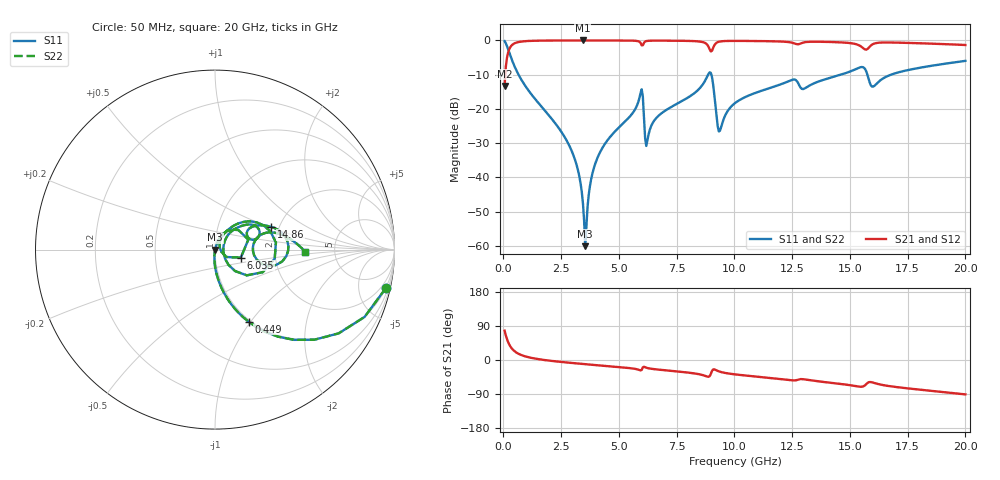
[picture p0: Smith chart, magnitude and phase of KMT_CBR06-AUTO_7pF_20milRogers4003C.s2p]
! Data measured by Modelithics Inc. support@modelithics.com 813-866-6335
! KEMET CBR06-AUTO 7pF, Pad Width= 0.851mm, Pad Length= 0.64mm, Pad Gap= 0.62mm, 20mil Rogers 4003C substrate Data, January 2022
# hz S ma R 50
! 2 Port Network Data from SP1.SP block
! freq  magS11  angS11  magS21  angS21  magS12  angS12  magS22  angS22
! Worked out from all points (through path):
!   401 points, 50 MHz to 20 GHz, reference 50 ohm
!   highest |S21| = -0.01 dB at 3.442 GHz (marker M1); lowest = -13.3 dB at 50 MHz (marker M2)
!   group delay of S21, straight-line fit = 14 ps
!   lowest |S11| = -60.1 dB at 3.541 GHz (marker M3), VSWR 1.00, Z = 50.1 - j0.0405 ohm
!   |S11| at or under -10 dB: 654 MHz to 8.861 GHz (8.207 GHz wide, 173 % of centre); 9.001 GHz to 14.6 GHz (5.601 GHz wide, 47.5 % of centre); 15.76 GHz to 16.78 GHz (1.024 GHz wide, 6.29 % of centre)
!   |S22| runs from -60.1 to -0.2 dB; largest |S21 - S12| = 0
!   S11 on the Smith chart (normalised r, x): 50 MHz: 0.98, -8.90; 449 MHz: 0.98, -0.98; 6.035 GHz: 1.33, -0.12; 14.86 GHz: 1.82, +0.52; 20 GHz: 3.02, -0.10
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5e7  0.9762 -12.7  0.2167 77.3  0.2167 77.3  0.9762 -12.7
4.49e8  0.4429 -65.0  0.896 24.9  0.896 24.9  0.4429 -65.0
2.793125e9  0.03186 -95.4  0.9985 -6.9  0.9985 -6.9  0.03186 -95.4
3.192125e9  0.01418 -95.5  0.9989 -9.2  0.9989 -9.2  0.01418 -95.5
3.391625e9  0.006126 -91.4  0.9989 -10.2  0.9989 -10.2  0.006126 -91.4
3.4415e9  0.004198 -87.4  0.9989 -10.5  0.9989 -10.5  0.004198 -87.4
3.54125e9  0.0009928 -24.0  0.9989 -11.0  0.9989 -11.0  0.0009928 -24.0
3.8405e9  0.01103 72.1  0.9988 -12.6  0.9988 -12.6  0.01103 72.1
4.189625e9  0.02361 72.9  0.9985 -14.4  0.9985 -14.4  0.02361 72.9
5.93525e9  0.1702 39.8  0.9219 -27.5  0.9219 -27.5  0.1702 39.8
6.035e9  0.1505 -17.3  0.8493 -19.0  0.8493 -19.0  0.1505 -17.3
6.2345e9  0.03489 44.0  0.9847 -21.2  0.9847 -21.2  0.03489 44.0
6.73325e9  0.08061 62.1  0.9932 -25.6  0.9932 -25.6  0.08061 62.1
8.92775e9  0.3419 6.7  0.7429 -42.7  0.7429 -42.7  0.3419 6.7
9.32675e9  0.04689 -6.1  0.9566 -29.9  0.9566 -29.9  0.04689 -6.1
1.0025e10  0.1216 48.4  0.9844 -37.9  0.9844 -37.9  0.1216 48.4
1.336662e10  0.2301 31.7  0.9569 -54.3  0.9569 -54.3  0.2301 31.7
1.486288e10  0.3378 22.0  0.9245 -65.2  0.9245 -65.2  0.3378 22.0
1.576062e10  0.3128 -16.9  0.7496 -60.6  0.7496 -60.6  0.3128 -16.9
1.601e10  0.2119 3.9  0.8873 -59.8  0.8873 -59.8  0.2119 3.9
1.670825e10  0.3096 17.9  0.9334 -68.9  0.9334 -68.9  0.3096 17.9
2e10  0.5029 -1.4  0.8575 -90.7  0.8575 -90.7  0.5029 -1.4
